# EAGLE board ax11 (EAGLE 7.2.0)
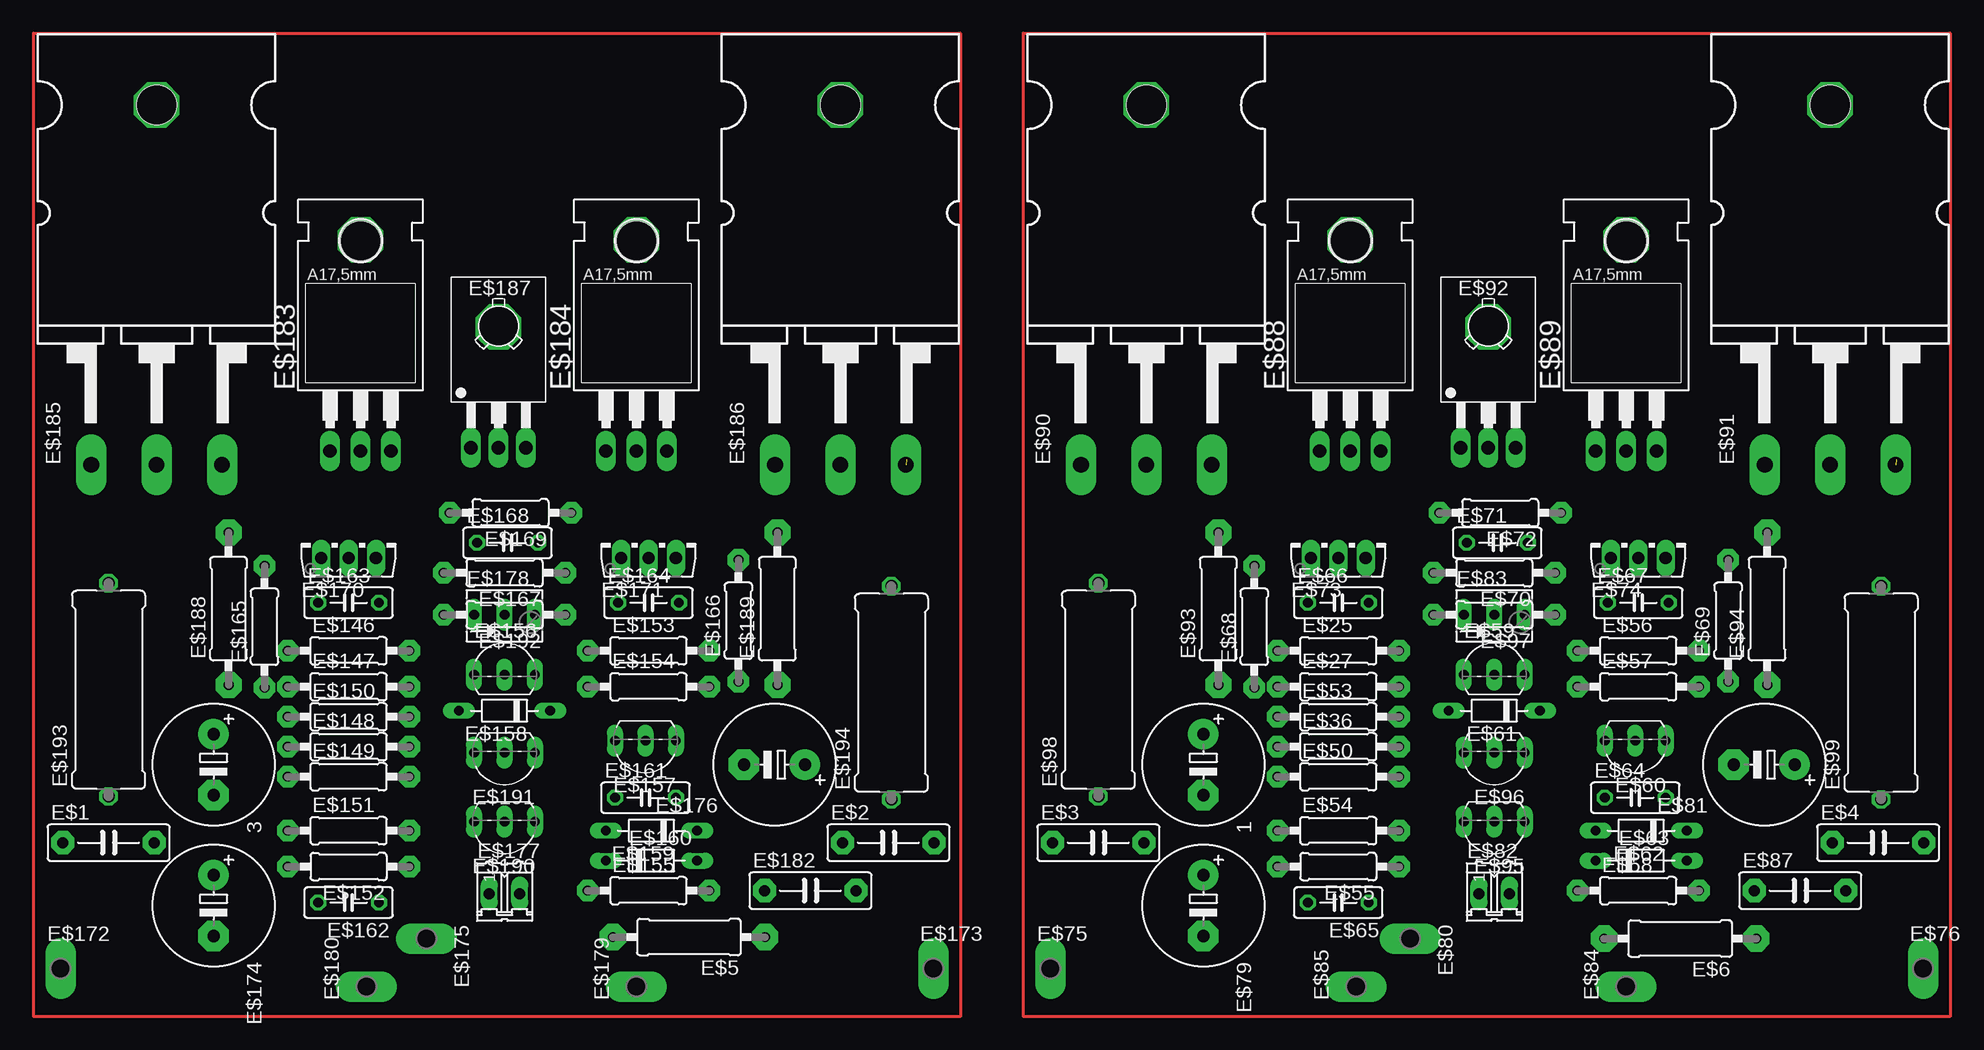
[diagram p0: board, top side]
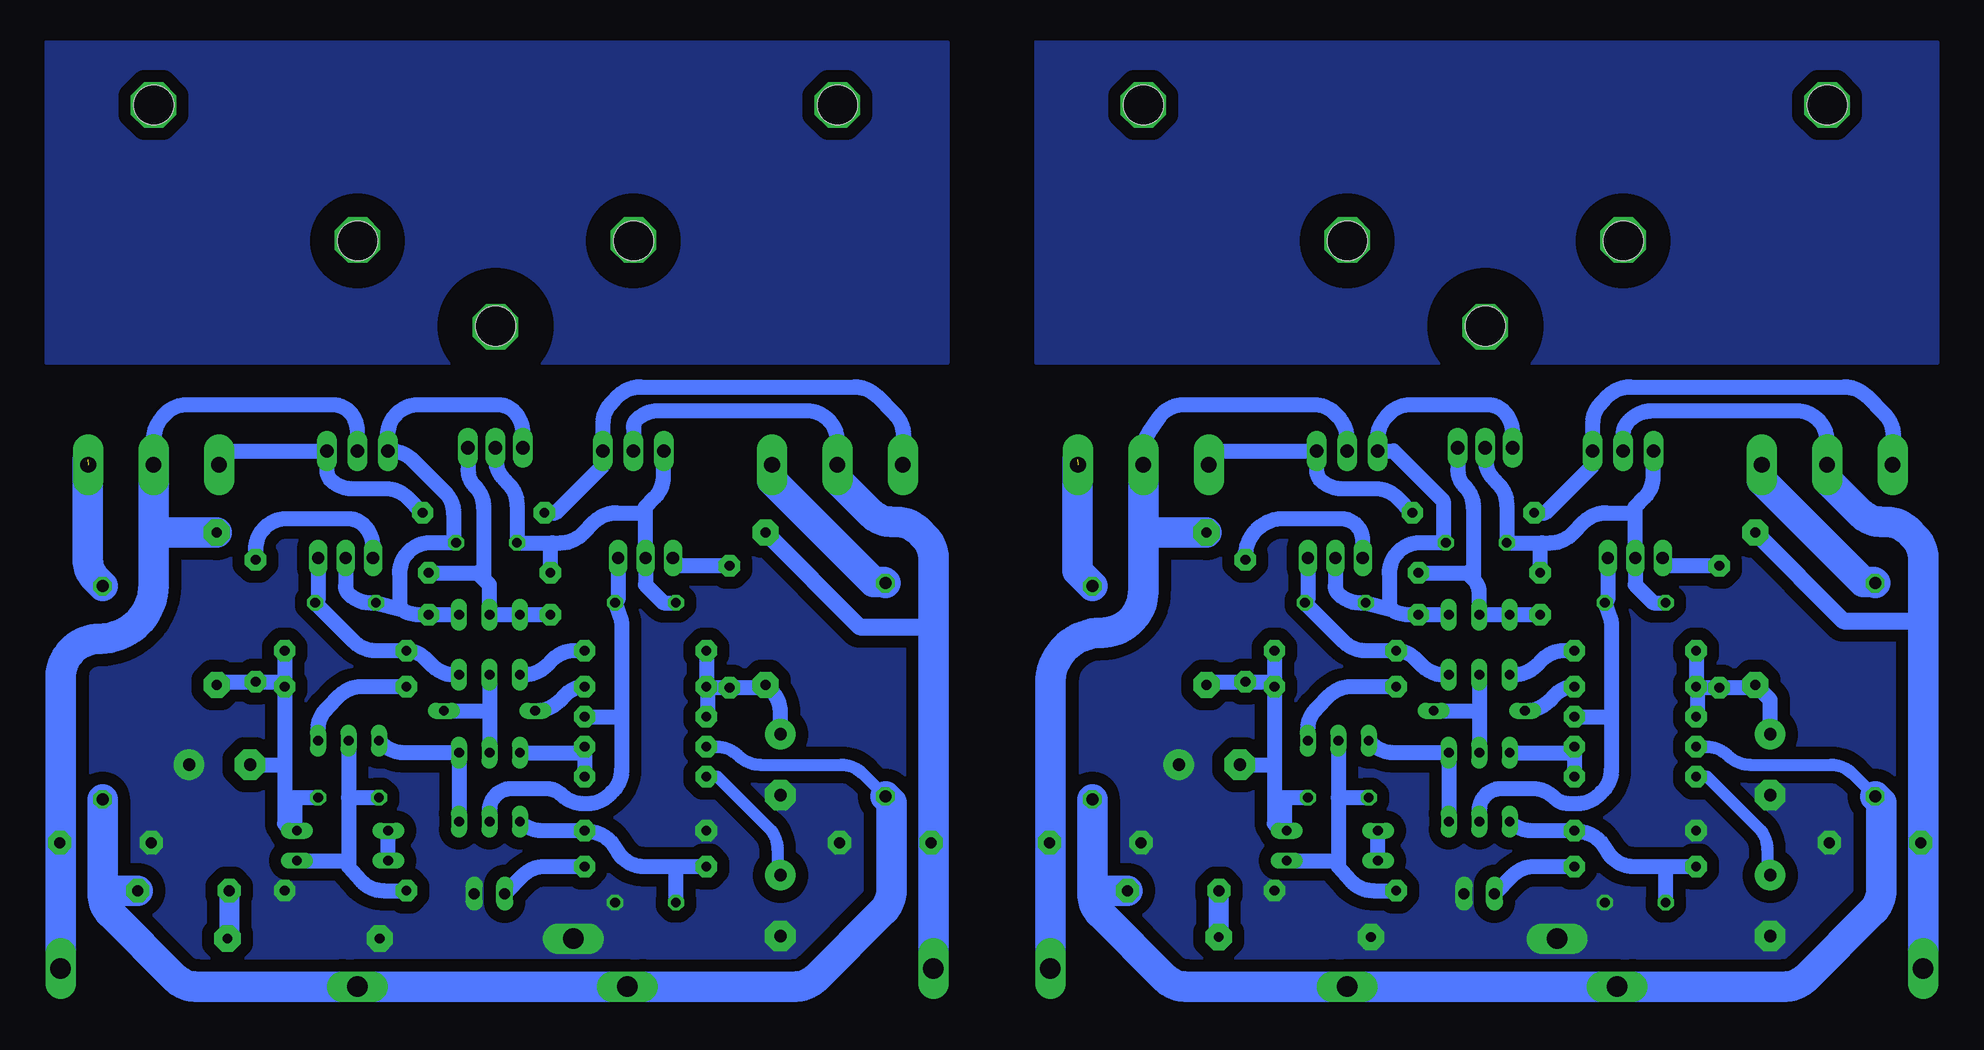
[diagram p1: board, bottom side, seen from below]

No outline drawn. Coordinates in mm, seen from the top.
Copper layers (1*16): Top 0.035mm / dielectric 1.5mm / Bottom 0.035mm
Design rules "default": minimum track width 10mil, minimum drill 24mil, track to track 8mil, track to pad 8mil, pad to pad 8mil, via to via 8mil, smd to smd 8mil, copper to edge 40mil, drill to drill 8mil, minimum pad ring 10mil, minimum via ring 8mil, stop-mask expansion 4mil, vias tented up to drill 0mil, thermal gap 10mil

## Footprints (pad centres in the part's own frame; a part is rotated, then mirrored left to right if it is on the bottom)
E5-10,5 = drill 1.016 pad 2.54: + -2.54,0 | drill 1.016 pad 2.54 octagon: - 2.54,0
C075-032X103 = drill 0.914 pad 1.93 octagon: 1 -3.81,0; 2 3.81,0
0309/12 = drill 0.813 pad 2.184 octagon: 1 -6.35,0; 2 6.35,0
0207/10 = drill 0.813 pad 1.778 octagon: 1 -5.08,0; 2 5.08,0
TO92 = drill 0.813 long: D -2.54,0; G 0,0; S 2.54,0
D-7.5 = drill 0.813 long: A 3.81,0; C -3.81,0
C050-025X075 = drill 0.813 octagon: 1 -2.54,0; 2 2.54,0
TO126AV = drill 1.016 long: B 2.286,-1.27; C 0,-1.27; E -2.286,-1.27
P1-17Y = drill 1.702 pad 2.121 long: TP 0,0
02P = drill 0.914 long: 1 -1.27,0; 2 1.27,0
B64Y = drill 0.813 long: A 2.54,0; E -2.54,0; S 0,0
TO220AB = drill 1.118 long: A1 -2.54,-6.35; A2 2.54,-6.35; C 0,-6.35 | hole 3.302: 0,11.176
TO264 = drill 1.3 pad 2.54 long: 1 -5.45,-30; 2 0,-30; 3 5.45,-30 | hole 3.3: 0,0
TO126 = drill 1.118 long: 1 -2.286,-5.08; 2 0,-5.08; 3 2.286,-5.08 | hole 3.302: 0,5.08
0617/17 = drill 1.016 octagon: 1 -8.89,0; 2 8.89,0

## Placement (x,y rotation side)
1  470u  [E5-10,5]  98.25,21.5 270 top
3  470u  [E5-10,5]  15.75,21.5 270 top
E$1  [C075-032X103]  7,15 0 top
E$2  [C075-032X103]  72,15 0 top
E$3  [C075-032X103]  89.5,15 0 top
E$4  [C075-032X103]  154.5,15 0 top
E$5  10  [0309/12]  55.38,7.12 180 top
E$6  10  [0309/12]  138,7 180 top
E$25  680  [0207/10]  109.5,31 0 top
E$27  680  [0207/10]  109.5,28 0 top
E$36  22k  [0207/10]  109.5,23 0 top
E$50  1k  [0207/10]  109.5,20.5 0 top
E$53  680  [0207/10]  109.5,25.5 0 top
E$54  22k  [0207/10]  109.5,16 0 top
E$55  2k2  [0207/10]  109.5,13 180 top
E$56  680  [0207/10]  134.5,31 0 top
E$57  180  [0207/10]  134.5,28 0 top
E$58  22k  [0207/10]  134.5,11 0 top
E$59  5401  [TO92]  122.5,29 0 top
E$60  5551  [TO92]  134.25,23.5 180 top
E$61  [D-7.5]  122.5,26 180 top
E$62  [D-7.5]  134.75,16 180 top
E$63  [D-7.5]  134.75,13.5 0 top
E$64  100n  [C050-025X075]  134.25,18.75 0 top
E$65  100p  [C050-025X075]  109.5,10 180 top
E$66  100p  [C050-025X075]  109.5,35 0 top
E$67  100p  [C050-025X075]  134.5,35 0 top
E$68  47  [0207/10]  102.5,33 90 top
E$69  47  [0207/10]  142,33.5 90 top
E$70  3k3  [0207/10]  122.5,37.5 180 top
E$71  100n  [C050-025X075]  122.75,40 0 top
E$72  220  [0207/10]  123,42.5 180 top
E$73  350  [TO126AV]  109.5,40 0 top
E$74  340  [TO126AV]  134.5,40 0 top
E$75  [P1-17Y]  85.5,4.5 0 top
E$76  [P1-17Y]  158.25,4.5 0 top
E$79  220u  [E5-10,5]  98.25,9.75 270 top
E$80  [P1-17Y]  115.5,7 270 top
E$81  470u  [E5-10,5]  145,21.5 180 top
E$82  [02P]  122.5,10.75 0 top
E$83  10k  [B64Y]  122.5,34 0 top
E$84  [P1-17Y]  133.5,3 90 top
E$85  [P1-17Y]  111,3 90 top
E$87  100n  [C075-032X103]  148,11 0 top
E$88  C4793  [TO220AB]  110.5,54 0 top
E$89  A1837  [TO220AB]  133.5,54 0 top
E$90  4281  [TO264]  93.5,76.5 0 top
E$91  4302  [TO264]  150.5,76.5 0 top
E$92  BD679  [TO126]  122,53 0 top
E$93  10  [0309/12]  99.5,34.5 90 top
E$94  10  [0309/12]  145.25,34.5 90 top
E$95  1775  [TO92]  122.5,16.75 180 top
E$96  1775  [TO92]  122.5,22.5 180 top
E$97  3k3  [0207/10]  122.5,34 180 top
E$98  [0617/17]  89.5,27.75 90 top
E$99  [0617/17]  154.75,27.5 90 top
E$146  680  [0207/10]  27,31 0 top
E$147  680  [0207/10]  27,28 0 top
E$148  22k  [0207/10]  27,23 0 top
E$149  1k  [0207/10]  27,20.5 0 top
E$150  680  [0207/10]  27,25.5 0 top
E$151  22k  [0207/10]  27,16 0 top
E$152  2k2  [0207/10]  27,13 180 top
E$153  680  [0207/10]  52,31 0 top
E$154  180  [0207/10]  52,28 0 top
E$155  22k  [0207/10]  52,11 0 top
E$156  5401  [TO92]  40,29 0 top
E$157  5551  [TO92]  51.75,23.5 180 top
E$158  [D-7.5]  40,26 180 top
E$159  [D-7.5]  52.25,16 180 top
E$160  [D-7.5]  52.25,13.5 0 top
E$161  100n  [C050-025X075]  51.75,18.75 0 top
E$162  100p  [C050-025X075]  27,10 180 top
E$163  100p  [C050-025X075]  27,35 0 top
E$164  100p  [C050-025X075]  52,35 0 top
E$165  47  [0207/10]  20,33 90 top
E$166  47  [0207/10]  59.5,33.5 90 top
E$167  3k3  [0207/10]  40,37.5 180 top
E$168  100n  [C050-025X075]  40.25,40 0 top
E$169  220  [0207/10]  40.5,42.5 180 top
E$170  350  [TO126AV]  27,40 0 top
E$171  340  [TO126AV]  52,40 0 top
E$172  [P1-17Y]  3,4.5 0 top
E$173  [P1-17Y]  75.75,4.5 0 top
E$174  220u  [E5-10,5]  15.75,9.75 270 top
E$175  [P1-17Y]  33.5,7 270 top
E$176  470u  [E5-10,5]  62.5,21.5 180 top
E$177  [02P]  40,10.75 0 top
E$178  10k  [B64Y]  40,34 0 top
E$179  [P1-17Y]  51,3 90 top
E$180  [P1-17Y]  28.5,3 90 top
E$182  100n  [C075-032X103]  65.5,11 0 top
E$183  C4793  [TO220AB]  28,54 0 top
E$184  A1837  [TO220AB]  51,54 0 top
E$185  4281  [TO264]  11,76.5 0 top
E$186  4302  [TO264]  68,76.5 0 top
E$187  BD679  [TO126]  39.5,53 0 top
E$188  10  [0309/12]  17,34.5 90 top
E$189  10  [0309/12]  62.75,34.5 90 top
E$190  1775  [TO92]  40,16.75 180 top
E$191  1775  [TO92]  40,22.5 180 top
E$192  3k3  [0207/10]  40,34 180 top
E$193  [0617/17]  7,27.75 90 top
E$194  [0617/17]  72.25,27.5 90 top

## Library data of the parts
1 3 E$1-E$4 E$25 E$27 E$36 E$50 E$53-E$58 E$64-E$72 E$79 E$81 E$87 E$97 E$146-E$155 E$161-E$169 E$174 E$176 E$182 E$192 = rcl
E$5 E$6 E$93 E$94 E$98 E$99 E$188 E$189 E$193 E$194 = resistor
E$59 E$60 E$95 E$96 E$156 E$157 E$190 E$191 = CBAndersen
E$61-E$63 E$88 E$89 E$158-E$160 E$183 E$184 = diode
E$73 E$74 E$170 E$171 = LME49810
E$75 E$76 E$80 E$84 E$85 E$172 E$173 E$175 E$179 E$180 = testpad
E$82 E$177 = con-amp-quick
E$83 E$178 = pot
E$90 E$91 E$185 E$186 = transistor-neu-to92
E$92 E$187 = ref-packages

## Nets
GND1: 1.- E$3.2 E$4.1 E$6.2 E$54.1 E$58.2 E$65.1 E$79.- E$80.TP E$81.+ E$82.2
GND3: 3.- E$1.2 E$2.1 E$5.2 E$151.1 E$155.2 E$162.1 E$174.- E$175.TP E$176.+ E$177.2
S$30: E$25.2 E$59.D
S$31: E$27.2 E$61.A
S$32: E$36.2 E$50.2 E$96.S
S$33: E$59.G E$61.C E$96.G
S$34: E$53.2 E$66.2 E$73.B E$95.G
S$35: E$54.2 E$55.2 E$65.2 E$95.S
S$36: 1.+ E$25.1 E$27.1 E$53.1 E$68.1 E$93.1
S$37: E$56.1 E$59.S E$67.2 E$74.B
S$38: E$57.1 E$60.D
S$39: E$58.1 E$60.G E$63.A E$64.1
S$40: E$62.A E$63.C
S$41: E$67.1 E$71.2 E$74.C E$83.A E$89.A1 E$92.1 E$97.1
S$42: E$68.2 E$73.E
S$43: E$56.2 E$57.2 E$62.C E$64.2 E$69.1 E$81.- E$94.1
S$44: E$69.2 E$74.E
S$45: E$70.1 E$83.E E$83.S E$92.3 E$97.2
S$46: E$66.1 E$70.2 E$71.1 E$73.C E$88.A1 E$92.2
S$47: E$72.2 E$88.A2 E$90.1
S$48: E$72.1 E$89.A2 E$91.1
S$49: E$4.2 E$76.TP E$89.C E$91.2 E$94.2
S$50: E$3.1 E$75.TP E$88.C E$90.2 E$93.2
S$51: E$90.3 E$98.2
S$52: E$91.3 E$99.2
S$53: E$50.1 E$79.+
S$54: E$55.1 E$82.1
S$55: E$36.1 E$84.TP E$85.TP E$87.2 E$98.1 E$99.1
S$56: E$6.1 E$87.1
S$57: E$60.S E$95.D E$96.D
S$93: E$146.2 E$156.D
S$94: E$147.2 E$158.A
S$95: E$148.2 E$149.2 E$191.S
S$96: E$156.G E$158.C E$191.G
S$97: E$150.2 E$163.2 E$170.B E$190.G
S$98: E$151.2 E$152.2 E$162.2 E$190.S
S$99: 3.+ E$146.1 E$147.1 E$150.1 E$165.1 E$188.1
S$100: E$153.1 E$156.S E$164.2 E$171.B
S$101: E$154.1 E$157.D
S$102: E$155.1 E$157.G E$160.A E$161.1
S$103: E$159.A E$160.C
S$104: E$164.1 E$168.2 E$171.C E$178.A E$184.A1 E$187.1 E$192.1
S$105: E$165.2 E$170.E
S$106: E$153.2 E$154.2 E$159.C E$161.2 E$166.1 E$176.- E$189.1
S$107: E$166.2 E$171.E
S$108: E$167.1 E$178.E E$178.S E$187.3 E$192.2
S$109: E$163.1 E$167.2 E$168.1 E$170.C E$183.A1 E$187.2
S$110: E$169.2 E$183.A2 E$185.1
S$111: E$169.1 E$184.A2 E$186.1
S$112: E$2.2 E$173.TP E$184.C E$186.2 E$189.2
S$113: E$1.1 E$172.TP E$183.C E$185.2 E$188.2
S$114: E$185.3 E$193.2
S$115: E$186.3 E$194.2
S$116: E$149.1 E$174.+
S$117: E$152.1 E$177.1
S$118: E$148.1 E$179.TP E$180.TP E$182.2 E$193.1 E$194.1
S$119: E$5.1 E$182.1
S$120: E$157.S E$190.D E$191.D

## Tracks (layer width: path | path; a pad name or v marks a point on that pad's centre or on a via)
GND1
  pour Bottom (isolate 1.016, no thermals): 86.5,44 157.5,44 157.5,2 86.5,2
GND3
  pour Bottom (isolate 1.016, no thermals): 4,44 75,44 75,2 4,2
S$30
  Bottom 1.27: E$25.2 115.45,31 arc-45 117.24,30.26 117.76,29.74 arc45 119.55,29 E$59.D
S$31
  Bottom 1.27: E$27.2 arc-45 116.15,27.35 116.76,26.74 arc45 118.55,26 E$61.A
S$32
  Bottom 1.27: E$36.2 114.58,22.5 | 114.58,22.5 E$50.2 | E$96.S 114.58,22.5
S$33
  Bottom 1.27: E$59.G 122.5,26 | 122.5,26 E$96.G | E$61.C 122.5,26
S$34
  Bottom 1.27: E$73.B 111.79,35.25 E$66.2 111.5,33.46 111.5,25.25 | 111.5,25.25 111.5,21.05 arc45 112.24,19.26 112.51,18.99 arc45 114.3,18.25 114.7,18.25 arc45 116.49,18.99 arc-45 117.72,19.5 120.7,19.5 arc-90 122.5,17.7 E$95.G | E$53.2 111.75,25.5 arc90 111.5,25.25
S$35
  Bottom 1.27: 107,13 109.63,13 arc57 111.75,14.14 112.17,14.78 arc-57 114.29,15.92 114.58,15.92 E$54.2 118.16,16 arc45 E$95.S | E$55.2 107,13 | E$65.2 106.96,12.96 107,13
S$36
  Bottom 1.27: E$25.1 E$27.1 104.34,27.92 | 104.34,27.92 E$68.1 99.5,27.92 E$93.1 98.99,27.64 arc45 98.25,25.85 1.+ | 104.34,27.92 104.34,25.58 E$53.1
S$37
  Bottom 1.27: E$74.B 136.79,35.25 E$67.2 133.78,31.74 arc-45 131.99,31 E$56.1 arc45 127.85,30.35 127.24,29.74 arc-45 125.45,29 E$59.S
S$38
  Bottom 1.27: E$57.1 133.2,28 arc-45 134.99,27.26 136.05,26.2 arc-45 136.79,24.41 E$60.D
S$39
  Bottom 1.27: E$60.G 134.25,18.75 | 134.25,18.75 134.25,13.5 | 134.25,13.5 134.25,13 133.26,11.87 arc-49 131.35,11 E$58.1 | E$63.A 134.25,13.5 | E$64.1 134.25,18.75
S$40
  Bottom 1.27: E$63.C E$62.A
S$41
  Bottom 1.27: E$74.C 134.5,36.36 arc-45 134.24,35.74 arc-45 132.45,35 E$67.1 130,34.5 | 130,34.5 130,37.45 arc45 129.26,39.24 129.24,39.26 arc45 127.45,40 E$71.2 125.5,40.04 125.5,42.45 arc-45 126.24,44.24 128.91,46.91 arc-45 130.7,47.65 E$89.A1 131,47.69 131,48.95 arc45 130.26,50.74 130.24,50.76 arc45 128.45,51.5 121.77,51.5 arc45 120.46,50.96 arc45 119.71,49.16 E$92.1 | E$83.A E$97.1 128.4,34 arc27 129.54,34.27 130,34.5
S$42
  Bottom 1.27: E$68.2 106.56,38.08 E$73.E
S$43
  Bottom 1.27: E$56.2 E$57.2 | E$57.2 140,28.42 E$69.1 145,28.42 E$94.1 | E$57.2 139.58,21.5 | 139.58,21.5 139.58,16.58 139,16 E$62.C 138.75,16.19 138.75,18.75 E$64.2 | E$81.- 139.58,21.5
S$44
  Bottom 1.27: E$74.E 132.21,39.66 arc-45 132.96,41.46 arc-45 134.27,42 139.45,42 arc-45 141.24,41.26 141.26,41.24 arc-45 142,39.45 E$69.2
S$45
  Bottom 1.27: E$70.1 123.5,37.5 123,37 | 123,37 122.5,36.5 E$83.S E$83.E E$97.2 | E$92.3 124.29,46.05 arc-45 123.74,44.74 arc45 123,42.95 123,37
S$46
  Bottom 1.016: 108,45 108,46.92
  Bottom 1.27: E$66.1 108,35 109.5,36.5 E$73.C 109.5,42.5 | 109.5,42.5 109.5,43 108.74,43.76 arc-45 108,45.55 108,46.92 107.96,46.96 E$88.A1 | E$92.2 122,47.05 arc-45 121.26,45.26 120.95,44.95 arc45 120.21,43.16 E$71.1 117.25,40 | 117.25,40 116.55,40 arc-45 114.76,40.74 113.74,41.76 arc45 111.95,42.5 109.5,42.5 | E$70.2 117.42,39.83 117.25,40
S$47
  Bottom 1.27: E$72.2 117,42.5 113,46.5 113,46.92 113.04,46.96 E$88.A2 113.04,49.91 arc45 112.3,51.7 111.74,52.26 arc45 109.95,53 92.05,53 arc45 90.26,52.26 88.74,50.74 arc45 88,48.95 88,46.55 arc90 E$90.1
S$48
  Bottom 1.27: E$72.1 129.34,43.76 arc-45 131.13,44.5 133.95,44.5 arc45 135.74,45.24 arc45 136.04,45.96 E$89.A2 144.4,47.65 E$91.1
S$49
  Bottom 1.27: E$91.2 150.5,48.65 arc37 149.99,50.18 149.76,50.48 arc53 147.73,51.5 135.53,51.5 arc56 133.93,50.64 arc34 133.5,49.23 E$89.C 133.5,46.96
  Bottom 1.422: E$4.2 158.25,15
  Bottom 2.54: E$76.TP 158.25,15 158.25,28.75 arc90 155,32 arc-90 150.5,36.5 150.5,40.5 | E$91.2 150.5,40.5 | E$94.2 150.15,40.85 arc-90 150.5,40.5
S$50
  Bottom 1.27: E$90.2 93.5,48.45 arc-45 94.24,50.24 94.26,50.26 arc-45 96.05,51 108.45,51 arc-45 110.24,50.26 arc-45 110.5,49.64 E$88.C 110.5,46.96 | 85.67,38.08 85.5,38.25
  Bottom 1.422: E$3.1 85.5,15 | E$93.2 91.65,33 85.5,33
  Bottom 2.54: E$90.2 93.5,45.25 90.74,42.49 arc-45 88.95,41.75 88.55,41.75 arc45 86.76,41.01 86.24,40.49 arc45 85.5,38.7 85.5,38.25 85.5,33 85.5,15 E$75.TP
S$51
  Bottom 2.54: E$90.3 98.95,45.2 90.5,36.75 89.61,36.75 E$98.2
S$52  (1 unrouted)
  Bottom 2.54: 156,46.95 156,38.69 arc-45 155.26,36.9 E$99.2
S$53
  Bottom 1.016: E$50.1 103.5,20.5 99.24,16.24 arc45 98.5,14.45 98.5,12.54 E$79.+
S$54
  Bottom 1.27: E$55.1 117.93,13 arc-45 119.72,12.26 E$82.1
S$55
  Bottom 1.016: E$36.1 103.55,23 arc45 101.76,22.26 101.74,22.24 arc-45 99.95,21.5 93.19,21.5 arc45 91.4,20.76 E$98.1
  Bottom 2.54: 154.75,11 154.75,10.8 arc-45 154.01,9.01 148.74,3.74 arc-45 146.95,3 E$84.TP E$85.TP 97.05,3 arc-45 95.26,3.74 89.74,9.26 arc-45 89,11.05 89,18.36 E$98.1 | E$99.1 154.75,11 | E$87.2 154.75,11
S$56
  Bottom 1.676: E$87.1 144.19,7.16 arc90 E$6.1
S$57
  Bottom 1.27: E$95.D E$96.D 129.66,22.5 arc45 131.45,23.24 E$60.S
S$58
  Top 0.254: 83.25,82.5 160.5,82.5 160.5,0.5 83.25,0.5 83.25,82.5
S$59  (via drill 1 pad 3.81)
  other vias: 93.5,76.5
S$60  (via drill 1 pad 3.81)
  other vias: 110.5,65.25
S$61  (via drill 1 pad 3.81)
  other vias: 122,58
S$62  (via drill 1 pad 3.81)
  other vias: 133.5,65.25
S$63  (via drill 1 pad 3.81)
  other vias: 150.5,76.5
S$64
  pour Bottom (isolate 1.016): 84.25,81.75 159.5,81.75 159.5,55 84.25,55
S$93
  Bottom 1.27: E$146.2 32.95,31 arc-45 34.74,30.26 35.26,29.74 arc45 37.05,29 E$156.D
S$94
  Bottom 1.27: E$147.2 arc-45 33.65,27.35 34.26,26.74 arc45 36.05,26 E$158.A
S$95
  Bottom 1.27: E$148.2 32.08,22.5 | 32.08,22.5 E$149.2 | E$191.S 32.08,22.5
S$96
  Bottom 1.27: E$156.G 40,26 | 40,26 E$191.G | E$158.C 40,26
S$97
  Bottom 1.27: E$170.B 29.29,35.25 E$163.2 29,33.46 29,25.25 | 29,25.25 29,21.05 arc45 29.74,19.26 30.01,18.99 arc45 31.8,18.25 32.53,18.25 arc45 33.76,18.76 arc-45 35.55,19.5 38.2,19.5 arc-90 40,17.7 E$190.G | E$150.2 29.25,25.5 arc90 29,25.25
S$98
  Bottom 1.27: 24.5,13 27.13,13 arc57 29.25,14.14 29.67,14.78 arc-57 31.79,15.92 32.08,15.92 E$151.2 35.66,16 arc45 E$190.S | E$152.2 24.5,13 | E$162.2 24.46,12.96 24.5,13
S$99
  Bottom 1.27: E$146.1 E$147.1 21.84,27.92 | 21.84,27.92 E$165.1 17,27.92 E$188.1 15.75,26.9 3.+ | 21.84,27.92 21.84,25.58 E$150.1
S$100
  Bottom 1.27: E$171.B 54.29,35.25 E$164.2 51.28,31.74 arc-45 49.49,31 E$153.1 arc45 45.35,30.35 44.74,29.74 arc-45 42.95,29 E$156.S
S$101
  Bottom 1.27: E$154.1 50.7,28 arc-45 52.49,27.26 53.55,26.2 arc-45 54.29,24.41 E$157.D
S$102
  Bottom 1.27: E$157.G 51.75,18.75 | 51.75,18.75 51.75,13.5 | 51.75,13.5 51.75,13 50.76,11.87 arc-49 48.85,11 E$155.1 | E$160.A 51.75,13.5 | E$161.1 51.75,18.75
S$103
  Bottom 1.27: E$160.C E$159.A
S$104
  Bottom 1.27: E$171.C 52,36.36 arc-45 51.74,35.74 arc-45 49.95,35 E$164.1 47.5,34.5 | 47.5,34.5 47.5,37.45 arc45 46.76,39.24 46.74,39.26 arc45 44.95,40 E$168.2 43,40.04 43,43.5 47.15,47.65 E$184.A1 48.5,47.69 48.5,48.65 arc37 47.99,50.18 47.76,50.48 arc53 45.73,51.5 39.27,51.5 arc45 37.96,50.96 arc45 37.21,49.16 E$187.1 | E$178.A E$192.1 45.9,34 arc27 47.04,34.27 47.5,34.5
S$105
  Bottom 1.27: E$165.2 24.06,38.08 E$170.E
S$106
  Bottom 1.27: E$153.2 E$154.2 | E$154.2 57.5,28.42 E$166.1 62.5,28.42 E$189.1 | E$154.2 57.08,21.5 | 57.08,21.5 57.08,16.58 56.5,16 E$159.C 56.25,16.19 56.25,18.75 E$161.2 | E$176.- 57.08,21.5
S$107
  Bottom 1.27: E$171.E 49.71,40.21 arc-90 51.5,42 56.58,42 arc-90 E$166.2
S$108
  Bottom 1.27: E$167.1 41,37.5 40.5,37 | 40.5,37 arc45 40,35.79 E$178.S E$178.E E$192.2 | E$187.3 41.79,46.05 arc-45 41.24,44.74 arc45 40.5,42.95 40.5,37
S$109
  Bottom 1.016: 25.5,45 25.5,46.92
  Bottom 1.27: E$187.2 39.5,47.05 arc-45 38.76,45.26 38.45,44.95 arc45 37.71,43.16 E$168.1 34.75,40 | E$163.1 25.5,35 27,36.5 E$170.C 27,42.5 | 27,42.5 27,43 26.24,43.76 arc-45 25.5,45.55 25.5,46.92 25.46,46.96 E$183.A1 | 34.75,40 34.05,40 arc-45 32.26,40.74 31.24,41.76 arc45 29.45,42.5 27,42.5 | E$167.2 34.92,39.83 34.75,40
S$110
  Bottom 1.27: E$169.2 34.5,42.5 30.5,46.5 30.5,46.92 30.54,46.96 E$183.A2 30.54,49.91 arc45 29.8,51.7 29.24,52.26 arc45 27.45,53 9.55,53 arc45 7.76,52.26 6.24,50.74 arc45 5.5,48.95 5.5,46.55 arc90 E$185.1
S$111
  Bottom 1.27: E$169.1 46.84,43.76 arc-45 48.63,44.5 51.45,44.5 arc45 53.24,45.24 arc45 53.54,45.96 E$184.A2 61.9,47.65 E$186.1
S$112
  Bottom 1.27: E$186.2 68,47.73 arc34 67.57,49.14 66.75,50.37 arc56 64.64,51.5 53.77,51.5 arc53 51.74,50.48 51.51,50.18 arc37 51,48.65 E$184.C 51,46.96
  Bottom 1.422: E$2.2 75.75,15
  Bottom 2.54: E$173.TP 75.75,15 75.75,28.22 arc90 71.5,32.5 arc-90 68,36 68,41 | E$186.2 68,41 | E$189.2 67.85,40.85 arc90 68,41
S$113
  Bottom 1.27: E$185.2 11,48.45 arc-45 11.74,50.24 11.76,50.26 arc-45 13.55,51 25.64,51 arc-56 27.75,49.87 arc-34 28,49.06 E$183.C 28,46.96 | 3.17,38.08 3,38.25
  Bottom 1.422: E$1.1 3,15 | E$188.2 9.65,33.5 3,33.5
  Bottom 2.54: E$185.2 11,45.25 8.24,42.49 arc-45 6.45,41.75 6.05,41.75 arc45 4.26,41.01 3.74,40.49 arc45 3,38.7 3,38.25 3,33.5 3,15 E$172.TP
S$114
  Bottom 2.54: E$185.3 16.45,45.2 8,36.75 7.11,36.75 E$193.2
S$115  (1 unrouted)
  Bottom 2.54: 73.5,46.95 73.5,37.64 E$194.2
S$116
  Bottom 1.016: E$149.1 21,20.5 16.74,16.24 arc45 16,14.45 16,12.54 E$174.+
S$117
  Bottom 1.27: E$152.1 35.43,13 arc-45 37.22,12.26 E$177.1
S$118
  Bottom 1.016: E$148.1 21.05,23 arc45 19.26,22.26 19.24,22.24 arc-45 17.45,21.5 10.69,21.5 arc45 8.9,20.76 E$193.1
  Bottom 2.54: E$193.1 6.5,18.36 6.5,11.05 arc45 7.24,9.26 12.76,3.74 arc45 14.55,3 E$180.TP E$179.TP 64.45,3 arc45 66.24,3.74 71.51,9.01 arc45 72.25,10.8 72.25,11 | E$194.1 72.25,11 | E$182.2 72.25,11
S$119
  Bottom 1.676: E$182.1 arc-90 61.73,10.96 E$5.1
S$120
  Bottom 1.27: E$190.D E$191.D 47.16,22.5 arc45 48.95,23.24 E$157.S
S$121
  Top 0.254: 0.75,82.5 78,82.5 78,0.5 0.75,0.5 0.75,82.5
S$122  (via drill 1 pad 3.81)
  other vias: 11,76.5
S$123  (via drill 1 pad 3.81)
  other vias: 28,65.25
S$124  (via drill 1 pad 3.81)
  other vias: 39.5,58
S$125  (via drill 1 pad 3.81)
  other vias: 51,65.25
S$126  (via drill 1 pad 3.81)
  other vias: 68,76.5
S$127
  pour Bottom (isolate 1.016): 1.75,81.75 77,81.75 77,55 1.75,55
